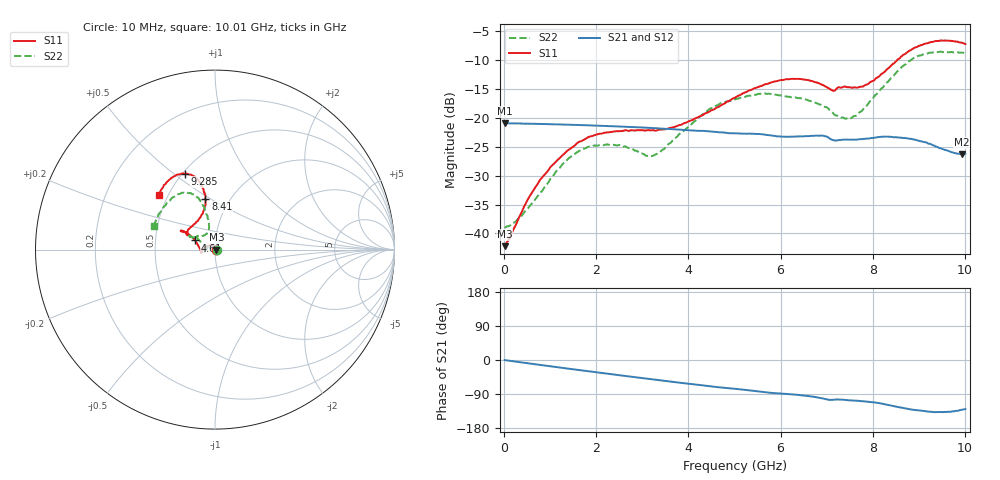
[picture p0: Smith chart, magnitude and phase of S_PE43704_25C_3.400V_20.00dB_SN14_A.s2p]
! Device ID: PE43704
! Dir: z:\PE43704\PE43704_Char_1_20130516\PE43704\AMB\3p400V\20p00dB
! Serial: 14
! Insertion: A
! Impedance: 50 ohm
! Temp: Amb
! VDD: 3.400V
! Attenuation Step: 20.00dB
! IDD: 1.140121e-01mA
#  Hz  S  RI  R  50
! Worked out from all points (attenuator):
!   401 points, 10 MHz to 10.01 GHz, reference 50 ohm
!   highest |S21| = -20.92 dB at 10 MHz (marker M1); lowest = -26.3 dB at 9.935 GHz (marker M2)
!   lowest |S11| = -42.2 dB at 10 MHz (marker M3), VSWR 1.02, Z = 50.8 + j0.0384 ohm
!   |S11| at or under -10 dB: start of sweep to 8.527 GHz
!   |S22| runs from -39.0 to -8.5 dB; largest |S21 - S12| = 0.00092
!   S11 on the Smith chart (normalised r, x): 10 MHz: 1.02, +0.00; 4.61 GHz: 0.80, +0.08; 8.41 GHz: 0.77, +0.47; 9.285 GHz: 0.52, +0.55; 10.01 GHz: 0.45, +0.34
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1e7  0.00775 0.000378  0.09 -0.000296  0.0899 -0.00032  0.0112 0.000291
3.35e8  0.00357 0.0136  0.089 -0.00887  0.089 -0.00881  0.00668 0.0119
8.1e8  -0.017 0.0248  0.0861 -0.0207  0.0862 -0.0206  -0.0124 0.0193
1.285e9  -0.0439 0.0199  0.0817 -0.0316  0.0817 -0.0316  -0.0386 0.0121
1.685e9  -0.0629 0.00716  0.0769 -0.0401  0.0769 -0.04  -0.0534 -0.00159
2.26e9  -0.074 -0.0115  0.0683 -0.0506  0.0683 -0.0506  -0.0565 -0.0157
3.11e9  -0.0766 -0.0163  0.0533 -0.0626  0.0534 -0.0625  -0.0469 -0.00238
3.36e9  -0.0786 -0.00991  0.0483 -0.0651  0.0484 -0.065  -0.0491 0.00768
4.61e9  -0.1117 0.0507  0.0241 -0.0716  0.0243 -0.0714  -0.108 0.0688
5.01e9  -0.1312 0.0722  0.0177 -0.0714  0.0179 -0.0714  -0.1264 0.0704
5.585e9  -0.1629 0.0962  0.00744 -0.0719  0.00759 -0.0717  -0.1418 0.0773
5.96e9  -0.1824 0.1052  0.00226 -0.0693  0.00242 -0.0691  -0.1408 0.0694
6.685e9  -0.1828 0.1002  -0.00792 -0.0694  -0.00797 -0.0692  -0.1219 0.066
7.135e9  -0.1498 0.0847  -0.0166 -0.0621  -0.0166 -0.0624  -0.0808 0.075
7.535e9  -0.1284 0.1299  -0.0187 -0.062  -0.0186 -0.0619  -0.045 0.0888
7.86e9  -0.0879 0.1728  -0.0223 -0.0623  -0.0222 -0.0623  -0.0337 0.122
8.36e9  -0.0525 0.2686  -0.0336 -0.06  -0.0333 -0.06  -0.0486 0.2069
8.41e9  -0.0531 0.282  -0.0347 -0.0591  -0.0347 -0.0591  -0.0547 0.2182
8.835e9  -0.0868 0.378  -0.0428 -0.0499  -0.0421 -0.0498  -0.1073 0.2984
9.285e9  -0.1667 0.4222  -0.0427 -0.0399  -0.0431 -0.0398  -0.1954 0.3101
9.935e9  -0.302 0.3296  -0.0319 -0.0363  -0.0325 -0.0365  -0.3307 0.1593
1.001e10  -0.3131 0.3043  -0.031 -0.038  -0.0314 -0.0379  -0.3404 0.1295
